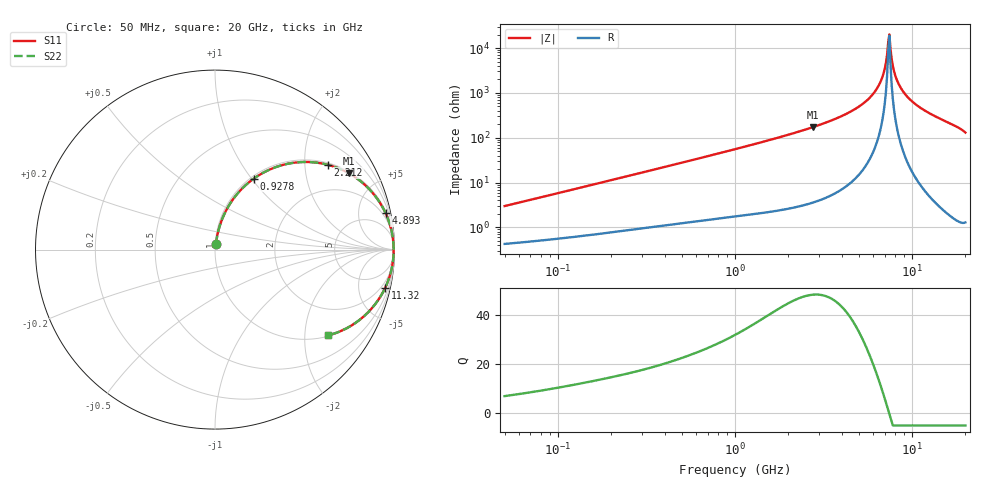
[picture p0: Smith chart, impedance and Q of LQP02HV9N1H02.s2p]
!Murata Part Number: LQP02HV9N1H02
!These Parameters are Measured in Series Mode Connection
!  o--[Z]--o
!Port1  Port2
!  o-------o
!Freq. Start=50[MHz] Stop=20[GHz], 401[Steps]
# Hz S RI R 50
!Freq.(Hz) S11(Real) S11(Imag) S21(Real) S21(Imag) S12(Real) S12(Imag) S22(Real) S22(Imag)
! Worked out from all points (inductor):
!   401 points, 50 MHz to 20 GHz, reference 50 ohm
!   read as one part in series: L = 9.34 nH near 51.52 MHz
!   highest Q = 48.1 at 2.769 GHz (marker M1), where L = 9.97 nH
!   self-resonance near 7.331 GHz
!   S11 on the Smith chart (normalised r, x): 50 MHz: 1.01, +0.06; 927.8 MHz: 1.03, +1.03; 2.212 GHz: 1.06, +2.62; 4.893 GHz: 1.27, +9.29; 11.32 GHz: 1.16, -8.93; 20 GHz: 1.03, -2.61
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5e7  0.00513 0.0294  0.9949 -0.0294  0.9949 -0.0294  0.00513 0.0294
1.364002e8  0.0123 0.0766  0.9877 -0.0766  0.9877 -0.0766  0.0123 0.0766
3.721004e8  0.0504 0.1946  0.9496 -0.1946  0.9496 -0.1946  0.0504 0.1946
9.278425e8  0.2165 0.3958  0.7835 -0.3958  0.7835 -0.3958  0.2165 0.3958
1e9  0.2422 0.4129  0.7578 -0.4129  0.7578 -0.4129  0.2422 0.4129
2.211938e9  0.6293 0.4723  0.3707 -0.4723  0.3707 -0.4723  0.6293 0.4723
2.728004e9  0.7387 0.4291  0.2613 -0.4291  0.2613 -0.4291  0.7387 0.4291
2.769174e9  0.7461 0.425  0.2539 -0.425  0.2539 -0.425  0.7461 0.425
4.89267e9  0.9504 0.2031  0.0496 -0.2031  0.0496 -0.2031  0.9504 0.2031
5.769027e9  0.9788 0.1244  0.0212 -0.1244  0.0212 -0.1244  0.9788 0.1244
6.406762e9  0.9896 0.0729  0.0104 -0.0729  0.0104 -0.0729  0.9896 0.0729
6.802353e9  0.9932 0.0432  0.00676 -0.0432  0.00676 -0.0432  0.9932 0.0432
7.009217e9  0.9944 0.0282  0.0056 -0.0282  0.0056 -0.0282  0.9944 0.0282
7.222371e9  0.9951 0.0133  0.0049 -0.0133  0.0049 -0.0133  0.9951 0.0133
7.442007e9  0.9953 -0.00172  0.00466 0.00172  0.00466 0.00172  0.9953 -0.00172
7.554318e9  0.9953 -0.00923  0.0047 0.00923  0.0047 0.00923  0.9953 -0.00923
8.020766e9  0.994 -0.0393  0.00604 0.0393  0.00604 0.0393  0.994 -0.0393
8.516016e9  0.9908 -0.0694  0.00924 0.0694  0.00924 0.0694  0.9908 -0.0694
9.600142e9  0.9786 -0.1296  0.0214 0.1296  0.0214 0.1296  0.9786 -0.1296
1.131968e10  0.9488 -0.2117  0.0512 0.2117  0.0512 0.2117  0.9488 -0.2117
1.597544e10  0.8245 -0.376  0.1755 0.376  0.1755 0.376  0.8245 -0.376
2e10  0.6282 -0.4783  0.3718 0.4783  0.3718 0.4783  0.6282 -0.4783
